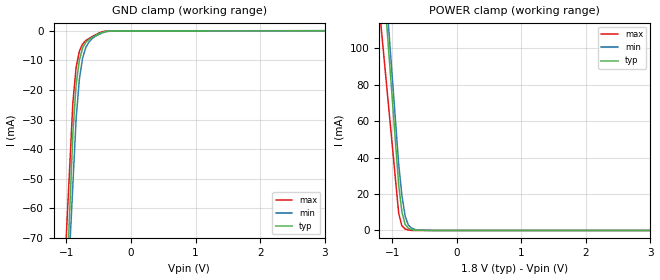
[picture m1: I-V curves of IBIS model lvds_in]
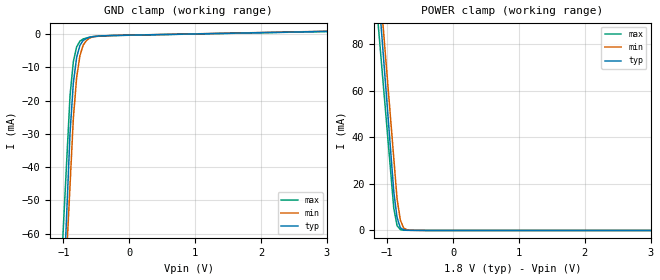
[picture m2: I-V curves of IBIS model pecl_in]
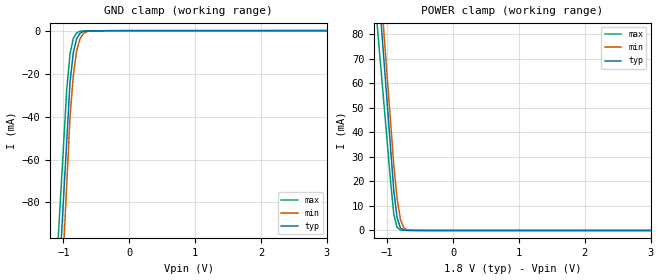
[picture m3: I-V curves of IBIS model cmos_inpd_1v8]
| Teraspeed Modeling Services.
| http://www.teraspeed.com
[IBIS Ver] 4.0
[File Name] dac3164.ibs
[File Rev] 1.0
[Date]   05-22-2013
[Notes]  Quality Check of this IBIS model: Model Passes IBIS Check. Model
   parses into ICX IS. Simulates with Hyperlynx.
   1. MIN TYP MAX information is based on Temperature and Voltage
   characteristics only.
   2. Package information extracted using Tektronix IConnect Software.
[Disclaimer]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
[Source]
| This model file was created by Teraspeed Consulting Group LLC
| (http://www.teraspeed.com/).
[Disclaimer]
| This product is designed as an aid for customers of Texas Instruments.
| No warranties, either expressed or implied, with respect to this third
| party software (if any) or with respect to its fitness for any
| particular purpose is claimed by Texas Instruments or the author. The
| software (if any) is provided solely on an "as is" basis. The entire
| risk as to its quality and performance is with the customer
[Copyright]
| (C) Copyright 2013 Texas Instruments Incorporated. All rights reserved.
| All other rights are reserved.
[Component] DAC3164
[Manufacturer] TI
[Package]
| variable   typ   min   max
R_pkg  1.766E-02   1.490E-02   2.060E-02
L_pkg  1.591E-09   1.340E-09   1.850E-09
C_pkg  4.418E-13   3.720E-13   5.150E-13
[Pin] signal_name  model_name  R_pin  L_pin C_pin
1   DACCLKP   pecl_in   2.060E-02   1.850E-09   5.150E-13
2   DACCLKN   pecl_in   1.970E-02   1.780E-09   4.930E-13
3   CLKVDD18   POWER   1.890E-02   1.700E-09   4.720E-13
4   ALIGNP   pecl_in   1.800E-02   1.620E-09   4.510E-13
5   ALIGNN   pecl_in   1.720E-02   1.550E-09   4.300E-13
6   SYNCP   lvds_in   1.640E-02   1.480E-09   4.100E-13
7   SYNCN   lvds_in   1.560E-02   1.410E-09   3.910E-13
8   VFUSE   POWER   1.490E-02   1.340E-09   3.720E-13
9   D11P   lvds_in   1.490E-02   1.340E-09   3.720E-13
10   D11N   lvds_in   1.560E-02   1.410E-09   3.910E-13
11   D10P   lvds_in   1.640E-02   1.480E-09   4.100E-13
12   D10N   lvds_in   1.720E-02   1.550E-09   4.300E-13
13   D9P   lvds_in   1.800E-02   1.620E-09   4.510E-13
14   D9N   lvds_in   1.890E-02   1.700E-09   4.720E-13
15   D8P   lvds_in   1.970E-02   1.780E-09   4.930E-13
16   D8N   lvds_in   2.060E-02   1.850E-09   5.150E-13
17   D7P   lvds_in   2.060E-02   1.850E-09   5.150E-13
18   D7N   lvds_in   1.970E-02   1.780E-09   4.930E-13
19   D6P   lvds_in   1.890E-02   1.700E-09   4.720E-13
20   D6N   lvds_in   1.800E-02   1.620E-09   4.510E-13
21   DIGVDD18   POWER   1.720E-02   1.550E-09   4.300E-13
22   D5P   lvds_in   1.640E-02   1.480E-09   4.100E-13
23   D5N   lvds_in   1.560E-02   1.410E-09   3.910E-13
24   DATACLKP   lvds_in   1.490E-02   1.340E-09   3.720E-13
25   DATACLKN   lvds_in   1.490E-02   1.340E-09   3.720E-13
26   D4P   lvds_in   1.560E-02   1.410E-09   3.910E-13
27   D4N   lvds_in   1.640E-02   1.480E-09   4.100E-13
28   VDD   POWER   1.720E-02   1.550E-09   4.300E-13
29   D3P   lvds_in   1.800E-02   1.620E-09   4.510E-13
30   D3N   lvds_in   1.890E-02   1.700E-09   4.720E-13
31   D2P   lvds_in   1.970E-02   1.780E-09   4.930E-13
32   D2N   lvds_in   2.060E-02   1.850E-09   5.150E-13
33   D1P   lvds_in   2.060E-02   1.850E-09   5.150E-13
34   D1N   lvds_in   1.970E-02   1.780E-09   4.930E-13
35   D0P   lvds_in   1.890E-02   1.700E-09   4.720E-13
36   D0N   lvds_in   1.800E-02   1.620E-09   4.510E-13
37   NC   NC   1.720E-02   1.550E-09   4.300E-13
38   NC   NC   1.640E-02   1.480E-09   4.100E-13
39   NC   NC   1.560E-02   1.410E-09   3.910E-13
40   NC   NC   1.490E-02   1.340E-09   3.720E-13
41   RESETB   cmos_inpu   1.490E-02   1.340E-09   3.720E-13
42   SDENB   cmos_inpu   1.560E-02   1.410E-09   3.910E-13
43   SCLK   cmos_inpd   1.640E-02   1.480E-09   4.100E-13
44   SDIO   cmos_io   1.720E-02   1.550E-09   4.300E-13
45   IOVDD   POWER   1.800E-02   1.620E-09   4.510E-13
46   SDO   cmos_out   1.890E-02   1.700E-09   4.720E-13
47   ALARM   cmos_out   1.970E-02   1.780E-09   4.930E-13
48   TXENABLE   cmos_inpd   2.060E-02   1.850E-09   5.150E-13
49   SLEEP   cmos_inpd   2.060E-02   1.850E-09   5.150E-13
50   VDDA18   POWER   1.970E-02   1.780E-09   4.930E-13
51   NC   NC   1.890E-02   1.700E-09   4.720E-13
52   NC   NC   1.800E-02   1.620E-09   4.510E-13
53   IOUTB1   term   1.720E-02   1.550E-09   4.300E-13
54   IOUTB2   term   1.640E-02   1.480E-09   4.100E-13
55   VDDA33   POWER   1.560E-02   1.410E-09   3.910E-13
56   VDDA33   POWER   1.490E-02   1.340E-09   3.720E-13
57   BIASJ   term   1.490E-02   1.340E-09   3.720E-13
58   EXTIO   term   1.560E-02   1.410E-09   3.910E-13
59   VDDA33   POWER   1.640E-02   1.480E-09   4.100E-13
60   IOUTA2   term   1.720E-02   1.550E-09   4.300E-13
61   IOUTA1   term   1.800E-02   1.620E-09   4.510E-13
62   NC   NC   1.890E-02   1.700E-09   4.720E-13
63   NC   NC   1.970E-02   1.780E-09   4.930E-13
64   VDDA18   POWER   2.060E-02   1.850E-09   5.150E-13
EP   GND   GND   0.00E+00   0.00E+00   0.00E+00
[Diff Pin] inv_pin vdiff tdelay_typ tdelay_min  tdelay_max
1   2   200mV   NA   NA   NA
4   5   200mV   NA   NA   NA
6   7   175mV   NA   NA   NA
9   10   175mV   NA   NA   NA
11   12   175mV   NA   NA   NA
13   14   175mV   NA   NA   NA
15   16   175mV   NA   NA   NA
17   18   175mV   NA   NA   NA
19   20   175mV   NA   NA   NA
22   23   175mV   NA   NA   NA
24   25   175mV   NA   NA   NA
26   27   175mV   NA   NA   NA
29   30   175mV   NA   NA   NA
31   32   175mV   NA   NA   NA
33   34   175mV   NA   NA   NA
35   36   175mV   NA   NA   NA
[Series Pin Mapping]   pin_2   model_name
6   7   110_Ohms
9   10   110_Ohms
11   12   110_Ohms
13   14   110_Ohms
15   16   110_Ohms
17   18   110_Ohms
19   20   110_Ohms
22   23   110_Ohms
24   25   110_Ohms
26   27   110_Ohms
29   30   110_Ohms
31   32   110_Ohms
33   34   110_Ohms
35   36   110_Ohms
[Model Selector]   cmos_inpu
cmos_inpu_1v8   1.8V cmos input with pullup
cmos_inpu_2v5   2.5V cmos input with pullup
cmos_inpu_3v3   3.3V cmos input with pullup
[Model Selector]   cmos_inpd
cmos_inpd_1v8   1.8V cmos input with pulldown
cmos_inpd_2v5   2.5V cmos input with pulldown
cmos_inpd_3v3   3.3V cmos input with pulldown
[Model Selector]   cmos_out
cmos_outpd_1v8  1.8V cmos output with pulldown
cmos_outpd_2v5  2.5V cmos output with pulldown
cmos_outpd_3v3  3.3V cmos output with pulldown
[Model Selector]   cmos_io
cmos_iopd_1v8   1.8V cmos IO with pulldown
cmos_iopd_2v5   2.5V cmos IO with pulldown
cmos_iopd_3v3   3.3V cmos IO with pulldown
[Model]  110_Ohms
Model_type Series
C_comp   0   0   0
[Voltage Range]  1.80   1.70   1.90
[Temperature Range]   25   85   -40
[R series]   110   85   135
[Model]  term
Model_type Terminator
C_comp   0   0   0
[Voltage Range]  3.30  3.00  3.60
[Temperature Range]   25   85   -40
| Models and submodels in the file (16): lvds_in (Input), pecl_in (Input), cmos_inpd_1v8 (Input), cmos_inpd_2v5 (Input), cmos_inpd_3v3 (Input), cmos_inpu_1v8 (Input), cmos_inpu_2v5 (Input), cmos_inpu_3v3 (Input), cmos_iopd_1v8 (I/O), cmos_iopd_2v5 (I/O), cmos_iopd_3v3 (I/O), cmos_outpd_1v8 (3-state), cmos_outpd_2v5 (3-state), cmos_outpd_3v3 (3-state), 110_Ohms (Series), term (Terminator)
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[Model] lvds_in
Model_type Input
Vinl = 1.12500V
Vinh = 1.27500V
C_comp 882.000fF 879.000fF 885.000fF
| variable typ   min   max
[Voltage Range] 1.80000V 1.70000V 1.90000V
[POWER Clamp Reference] 1.80000V 1.70000V 1.90000V
[GND Clamp Reference] 0.00000V 0.00000V 0.00000V
[Temperature Range]   25   85   -40
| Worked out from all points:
|   GND clamp passes 1 mA (typ) near -0.50 V on its own axis
|   POWER clamp passes 1 mA (typ) near -0.73 V on its own axis
[GND Clamp]
-1.8V     -516.4mA   -450.7mA   -422.4mA
-900mV    -34.53mA   -51.9mA    -24.17mA
-850mV    -18.27mA   -29.75mA   -12.3mA
-800mV    -9.904mA   -16.43mA   -6.903mA
-750mV    -5.838mA   -9.264mA   -4.466mA
-700mV    -3.875mA   -5.596mA   -3.283mA
-650mV    -2.888mA   -3.778mA   -2.59mA
-600mV    -2.244mA   -2.599mA   -1.898mA
-500mV    -957.3uA   -1.28mA    -772.7uA
-400mV    -203.4uA   -359.4uA   -116.6uA
-350mV    -165.3uA   -129.6uA   -92.98uA
3.6V      34.64uA    93.6uA     41.96uA
[POWER Clamp]
-1.8V     453.5mA    469.3mA    347.9mA
-1V       72.49mA    84.47mA    46.91mA
-900mV    24.87mA    36.36mA    9.282mA
-850mV    10.07mA    19.19mA    2.491mA
-800mV    3.31mA     7.858mA    827.6uA
-750mV    1.232mA    2.889mA    239.1uA
-700mV    479.2uA    1.326mA    35.61uA
-600mV    111.6uA    154.4uA    26.71uA
3.6V      0A         0A         0A
[Model] pecl_in
Model_type Input
Vinl = 400.000mV
Vinh = 1.00000V
C_comp 885.000fF 863.000fF 907.000fF
| variable typ   min   max
[Voltage Range] 1.80000V 1.70000V 1.90000V
[POWER Clamp Reference] 1.80000V 1.70000V 1.90000V
[GND Clamp Reference] 0.00000V 0.00000V 0.00000V
[Temperature Range]   25   85   -40
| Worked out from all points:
|   GND clamp passes 1 mA (typ) near -0.60 V on its own axis
|   POWER clamp passes 1 mA (typ) near -0.79 V on its own axis
[GND Clamp]
-1.8V     -461.7mA   -406.1mA   -369.2mA
-900mV    -29.73mA   -45.46mA   -18.51mA
-850mV    -14.79mA   -25.42mA   -8.318mA
-800mV    -7.02mA    -13.11mA   -3.88mA
-750mV    -3.412mA   -6.512mA   -2.125mA
-700mV    -1.892mA   -3.308mA   -1.472mA
-650mV    -1.305mA   -1.906mA   -1.2mA
-600mV    -985.7uA   -1.18mA    -928.5uA
-500mV    -673.3uA   -672.2uA   -695.2uA
3.6V      1.026mA    1.084mA    988.3uA
[POWER Clamp]
-1.8V     348.4mA    345.8mA    309.2mA
-1V       53.54mA    65.95mA    42.84mA
-900mV    16.68mA    30.97mA    9.541mA
-850mV    5.464mA    13.48mA    2.063mA
-800mV    1.156mA    4.432mA    378.8uA
-750mV    269.4uA    1.018mA    100.7uA
-700mV    89.55uA    281.3uA    88.83uA
-650mV    76.75uA    76.37uA    76.99uA
3.6V      0A         0A         0A
[Model] cmos_inpd_1v8
Model_type Input
Vinl = 450.000mV
Vinh = 1.08000V
C_comp 865.000fF 865.000fF 865.000fF
| variable typ   min   max
[Voltage Range] 1.80000V 1.71000V 1.89000V
[POWER Clamp Reference] 1.80000V 1.71000V 1.89000V
[GND Clamp Reference] 0.00000V 0.00000V 0.00000V
[Temperature Range]   25   85   -40
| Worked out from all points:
|   GND clamp passes 1 mA (typ) near -0.73 V on its own axis
|   POWER clamp passes 1 mA (typ) near -0.80 V on its own axis
[GND Clamp]
-1.8V     -518.4mA   -605mA     -482.8mA
-950mV    -51.38mA   -71.58mA   -27.3mA
-900mV    -23.91mA   -40.2mA    -10.85mA
-850mV    -10.2mA    -20.83mA   -3.517mA
-800mV    -3.824mA   -9.382mA   -1.017mA
-750mV    -1.288mA   -3.836mA   -302.4uA
-700mV    -411.3uA   -1.472mA   -137.1uA
-600mV    -138.8uA   -193.7uA   -104uA
3.6V      23.98uA    36.49uA    15.85uA
[POWER Clamp]
-1.8V     335.8mA    350.6mA    286.9mA
-1V       51.75mA    62.67mA    36.13mA
-950mV    34mA       44.67mA    20.46mA
-900mV    16.24mA    26.67mA    6.636mA
-850mV    5.335mA    13.03mA    1.244mA
-800mV    1.085mA    4.618mA    196.7uA
-750mV    194.4uA    1.173mA    48.92uA
-700mV    43.28uA    273.2uA    43.03uA
-650mV    37.1uA     62.6uA     37.14uA
3.6V      0A         0A         0A
